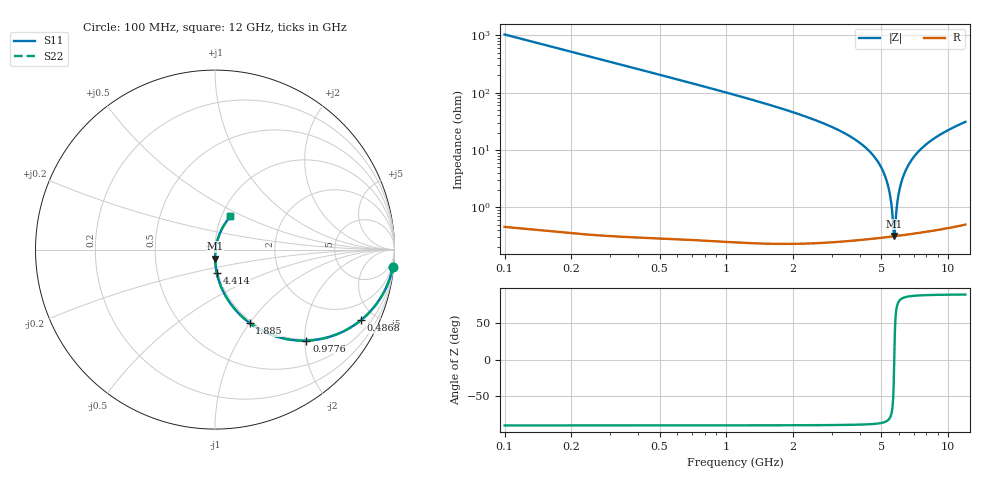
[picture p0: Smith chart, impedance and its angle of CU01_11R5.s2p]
! S-parameter model data by Modelithics Inc. support@modelithics.com 813-866-6335 Tampa FL USA
! S-Parameter data specifications:
! Substrate: 20-mil Rogers, substrate thickness, H=0.508mm, Dielectric constant, Er=3.75
! PCB Mounting Pad Footprint: Pad width, PadW=0.35mm , Pad length, PadL=0.30mm , Pad gap, PadG (edge-to-edge)=0.25mm , Reference planes=0.85mm apart
! Created Tue May  8 14:01:25 2018
# hz S ma R 50
! 2 Port Network Data from SP1.SP block
! freq  magS11  angS11  magS21  angS21  magS12  angS12  magS22  angS22
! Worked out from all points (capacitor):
!   801 points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, 100 MHz to 12 GHz, reference 50 ohm
!   read as one part in series: C = 1.54 pF near 159.5 MHz
!   lowest |Z| = 315 mohm at 5.723 GHz (marker M1)
!   series resonance near 5.729 GHz, so ESL is about 500 pH
!   S11 on the Smith chart (normalised r, x): 100 MHz: 1, -20; 486.8 MHz: 0.97, -4.16; 977.6 MHz: 0.97, -2.04; 1.885 GHz: 0.97, -1.00; 4.414 GHz: 0.99, -0.27; 12 GHz: 1.10, +0.42
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1e8  0.9953 -5.6  0.09623 84.4  0.09623 84.4  0.9953 -5.6
2.785e8  0.9653 -15.4  0.2603 74.6  0.2603 74.6  0.9653 -15.4
4.8675e8  0.9036 -25.8  0.4272 64.2  0.4272 64.2  0.9036 -25.8
9.77625e8  0.7191 -44.9  0.6932 45.0  0.6932 45.0  0.7191 -44.9
1.394125e9  0.5789 -55.8  0.8134 34.0  0.8134 34.0  0.5789 -55.8
1.885e9  0.4516 -64.8  0.8902 25.0  0.8902 25.0  0.4516 -64.8
2.09325e9  0.408 -67.7  0.9109 22.0  0.9109 22.0  0.408 -67.7
4.071625e9  0.1596 -83.9  0.9845 5.2  0.9845 5.2  0.1596 -83.9
4.41375e9  0.1329 -85.6  0.9883 3.3  0.9883 3.3  0.1329 -85.6
5.72275e9  0.04969 -89.3  0.9956 -2.8  0.9956 -2.8  0.04969 -89.3
6.05e9  0.0322 -88.5  0.9962 -4.1  0.9962 -4.1  0.0322 -88.5
6.392125e9  0.01503 -83.0  0.9965 -5.5  0.9965 -5.5  0.01503 -83.0
6.511125e9  0.009434 -75.6  0.9966 -5.9  0.9966 -5.9  0.009434 -75.6
6.645e9  0.004091 -42.3  0.9966 -6.4  0.9966 -6.4  0.004091 -42.3
6.7045e9  0.003357 0.7  0.9966 -6.6  0.9966 -6.6  0.003357 0.7
6.9425e9  0.01201 66.1  0.9964 -7.5  0.9964 -7.5  0.01201 66.1
7.165625e9  0.0219 72.6  0.9962 -8.3  0.9962 -8.3  0.0219 72.6
7.522625e9  0.03745 75.0  0.9956 -9.6  0.9956 -9.6  0.03745 75.0
8.04325e9  0.05923 75.1  0.9944 -11.3  0.9944 -11.3  0.05923 75.1
8.87625e9  0.0922 73.5  0.9917 -14.0  0.9917 -14.0  0.0922 73.5
1.002162e10  0.1348 70.6  0.9865 -17.6  0.9865 -17.6  0.1348 70.6
1.2e10  0.2036 65.1  0.974 -23.6  0.974 -23.6  0.2036 65.1
